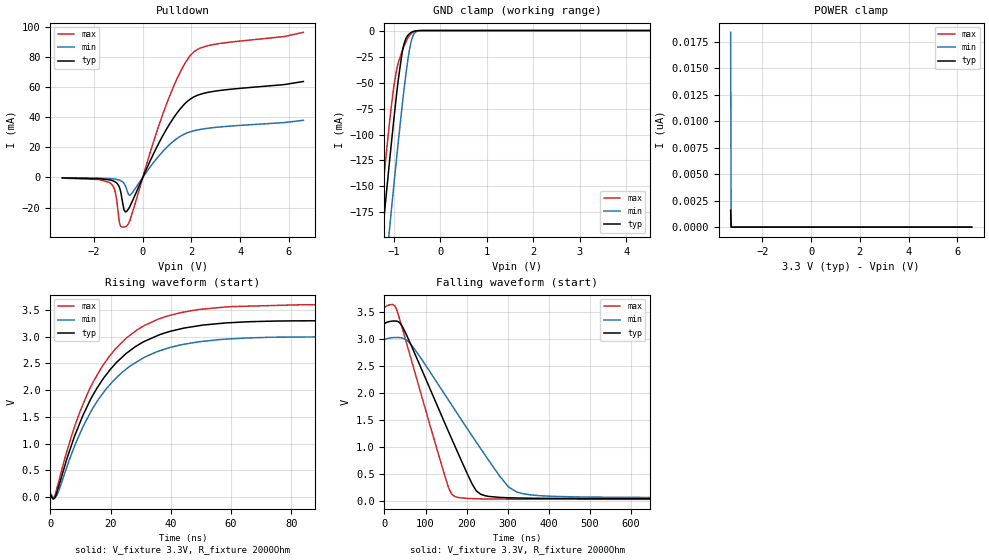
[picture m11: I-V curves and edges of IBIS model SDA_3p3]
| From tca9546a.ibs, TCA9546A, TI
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|   Model
[Model]   SDA_3p3
Model_type   I/O_open_drain
Polarity   Non-Inverting
Enable   Active-Low
Vinl = 0.99
Vinh = 2.31
Vmeas = 1.65
Vref = 3.3
Cref = 1pF
Rref = 2000
|   typ   min   max
C_comp   3.666pF   3.611pF   3.839pF
[Voltage Range]   3.3   3   3.6
[Temperature Range]   27   125   -40
[Pullup Reference]   3.3   3   3.6
[Pulldown Reference]   -0   -0   -0
[Power Clamp Reference]   3.3   3   3.6
[GND Clamp Reference]   -0   -0   -0
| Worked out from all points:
|   slope of the pulldown table from 0 to 0.495 V, typ, clamps not added: 28.3 ohm
|   GND clamp passes 1 mA (typ) near -0.58 V on its own axis
|   falling waveform, V_fixture 3.3V, R_fixture 2000Ohm: 20-80 % time 112ns typ, 154ns min, 80.7ns max; typ from 3.3 V to 0.044 V
|   rising waveform, V_fixture 3.3V, R_fixture 2000Ohm: 20-80 % time 19.1ns typ, 19.6ns min, 18.8ns max; typ from 0.044 V to 3.3 V
[Pulldown]
|   Voltage   I(typ)   I(min)   I(max)
-3.3V     -309.5uA   -173.9uA   -455.2uA
-1.32V    -1.754mA   -775.7uA   -3.815mA
-1.122V   -3.034mA   -1.128mA   -10.06mA
-943.8mV  -7.212mA   -1.833mA   -30.74mA
-765.6mV  -21.71mA   -4.031mA   -32.93mA
-686.4mV  -22.76mA   -6.677mA   -32.57mA
-488.4mV  -17.92mA   -11.34mA   -26.62mA
976.8mV   32.21mA    19.91mA    48.89mA
1.531V    45.46mA    27.28mA    69.86mA
1.947V    52.1mA     30.37mA    81.04mA
2.779V    56.89mA    32.93mA    88mA
6.59V     63.82mA    38.04mA    96.52mA
[GND Clamp]
|   Voltage   I(typ)   I(min)   I(max)
-3.3V     -1.2A      -1.263A    -1.161A
-1.379V   -260mA     -325.8mA   -219.2mA
-1.3V     -222.5mA   -288.3mA   -182mA
-1.241V   -194.7mA   -260.4mA   -154.6mA
-1.092V   -126.7mA   -191.6mA   -89.18mA
-1.013V   -91.93mA   -155.7mA   -58.83mA
-943.8mV  -63.18mA   -124.9mA   -39.09mA
-825mV    -22.64mA   -74.72mA   -20.4mA
-696.3mV  -4.717mA   -28.15mA   -7.384mA
-607.2mV  -1.408mA   -7.763mA   -2.263mA
-409.2mV  -27.92uA   -84.77uA   -29.5uA
6.59V     0A         0A         0A
[POWER Clamp]
|   Voltage   I(typ)   I(min)   I(max)
-3.3V     1.595nA    18.37nA    871.4pA
-3.28V    0A         0A         0A
-3.27V    0A         0A         0A
6.59V     0A         0A         0A
[Ramp]
R_load = 2000
|   typ   min   max
dV/dt_r   1.95384/1.91058e-08   1.76255/1.96429e-08   2.14095/1.87728e-08
dV/dt_f   1.95384/1.11585e-07   1.76256/1.53647e-07   2.14095/8.0701e-08
[Falling Waveform]
V_fixture = 3.3V
V_fixture_min = 3V
V_fixture_max = 3.6V
R_fixture = 2000Ohm
C_fixture = 0F
|   Time   V(typ)   V(min)   V(max)
0s        3.3V       3V         3.6V
28.87ns   3.335V     3.031V     3.562V
65.08ns   2.885V     2.897V     2.625V
148.1ns   1.42V      1.96V      435mV
171.3ns   1.02V      1.691V     84.36mV
212.9ns   321mV      1.211V     45.19mV
233.5ns   127.6mV    977.9mV    40.88mV
301.1ns   60.79mV    264.2mV    35.32mV
337.4ns   54.45mV    135mV      34.46mV
1us       43.59mV    62.39mV    31.75mV
[Rising Waveform]
V_fixture = 3.3V
V_fixture_min = 3V
V_fixture_max = 3.6V
R_fixture = 2000Ohm
C_fixture = 0F
|   Time   V(typ)   V(min)   V(max)
0s        43.59mV    62.4mV     31.75mV
1.064ns   -31mV      -2.856mV   -33.16mV
2.187ns   87.52mV    33.71mV    163.1mV
7.286ns   1.013V     840mV      1.185V
12.23ns   1.692V     1.464V     1.918V
16.73ns   2.141V     1.887V     2.395V
21.83ns   2.507V     2.224V     2.783V
35.8ns    3.024V     2.725V     3.325V
58.49ns   3.257V     2.953V     3.555V
1us       3.3V       3V         3.6V
